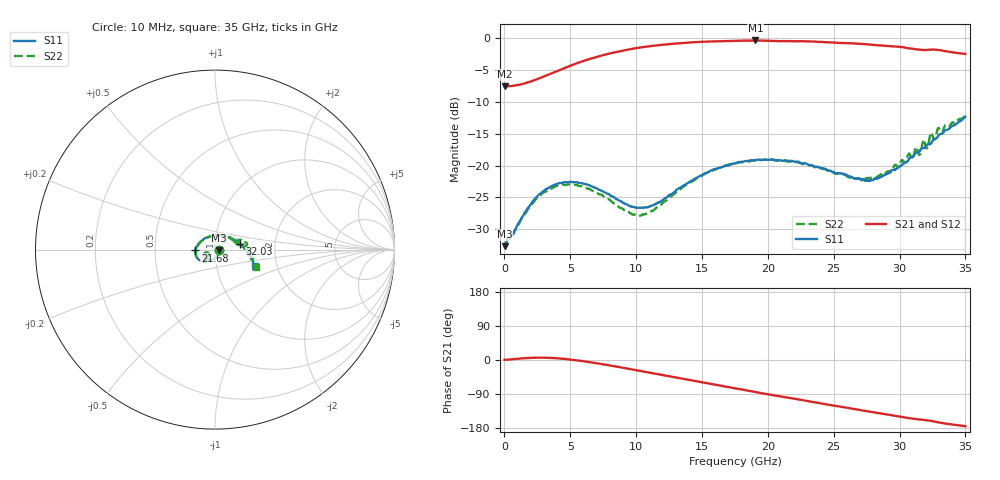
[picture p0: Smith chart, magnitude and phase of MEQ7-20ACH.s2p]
! MARKI MICROWAVE INC.
! Email:  support@markimicrowave.com  Phone:  408-778-4200
! Model Number:  MEQ7-20ACH  Date:  6/18
! Filename:		MEQ7-20ACH.S2P  Version: 1.0
! Description:  2-port S-parameter data for chip equalizer
! Features:		Low Insertion Loss, Excellent Return Loss
! Frequency Measured: 	10 MHz to 35 GHz
!S2P File: Measurements: S11, S21, S12, S22:
# Hz S  dB  R 50
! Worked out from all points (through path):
!   1601 points, 10 MHz to 35 GHz, reference 50 ohm
!   highest |S21| = -0.36 dB at 19.06 GHz (marker M1); lowest = -7.6 dB at 10 MHz (marker M2)
!   group delay of S21, straight-line fit = 16 ps
!   lowest |S11| = -32.6 dB at 10 MHz (marker M3), VSWR 1.05, Z = 52.4 - j0.332 ohm
!   |S11| at or under -10 dB: start of sweep to end of sweep
!   |S22| runs from -32.5 to -12.1 dB; largest |S21 - S12| = 0.01
!   S11 on the Smith chart (normalised r, x): 10 MHz: 1.05, -0.01; 21.68 GHz: 0.80, -0.01; 32.03 GHz: 1.32, +0.08; 35 GHz: 1.54, -0.30
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1e7  -32.65 -7.8  -7.57 0.8  -7.52 -0.0  -32.55 -2.7
2.677988e9  -24.44 -105.8  -6.27 6.2  -6.27 6.2  -24.77 -105.9
4.340012e9  -22.70 -133.4  -4.86 3.6  -4.86 3.6  -23.00 -134.3
5.848956e9  -22.77 -150.3  -3.68 -2.5  -3.68 -2.5  -23.24 -151.8
7.904619e9  -24.46 -161.5  -2.44 -13.7  -2.43 -13.8  -25.29 -162.5
9.741594e9  -26.50 -153.7  -1.66 -25.2  -1.66 -25.2  -27.68 -151.9
1.072569e10  -26.58 -143.0  -1.34 -31.5  -1.33 -31.5  -27.58 -138.1
1.168791e10  -25.80 -135.4  -1.10 -37.8  -1.09 -37.7  -26.44 -128.4
1.472767e10  -21.75 -131.2  -0.60 -57.3  -0.60 -57.3  -21.81 -127.7
1.7505e10  -19.64 -145.7  -0.42 -74.7  -0.42 -74.9  -19.66 -143.3
1.905768e10  -19.14 -156.2  -0.36 -84.5  -0.37 -84.4  -19.23 -154.0
2.168193e10  -19.25 -177.4  -0.46 -100.3  -0.48 -100.7  -19.37 -175.7
2.334396e10  -19.95 166.8  -0.53 -110.4  -0.51 -110.2  -20.04 167.1
2.717099e10  -22.19 108.2  -0.89 -133.1  -0.90 -132.9  -22.28 106.2
2.918291e10  -21.18 62.8  -1.23 -144.4  -1.20 -144.9  -20.89 62.6
3.123858e10  -17.99 24.3  -1.74 -155.8  -1.80 -155.7  -17.12 21.1
3.152287e10  -17.73 19.9  -1.80 -156.9  -1.84 -156.7  -18.32 18.9
3.182903e10  -17.27 12.7  -1.87 -158.0  -1.85 -157.7  -15.91 17.3
3.202585e10  -16.95 12.3  -1.85 -158.8  -1.82 -158.6  -17.20 18.2
3.237575e10  -16.57 6.8  -1.79 -160.6  -1.75 -160.4  -14.86 9.2
3.296621e10  -15.28 0.3  -1.85 -164.6  -1.79 -164.9  -14.08 2.1
3.5e10  -12.33 -22.2  -2.48 -174.6  -2.50 -174.3  -12.07 -23.5
